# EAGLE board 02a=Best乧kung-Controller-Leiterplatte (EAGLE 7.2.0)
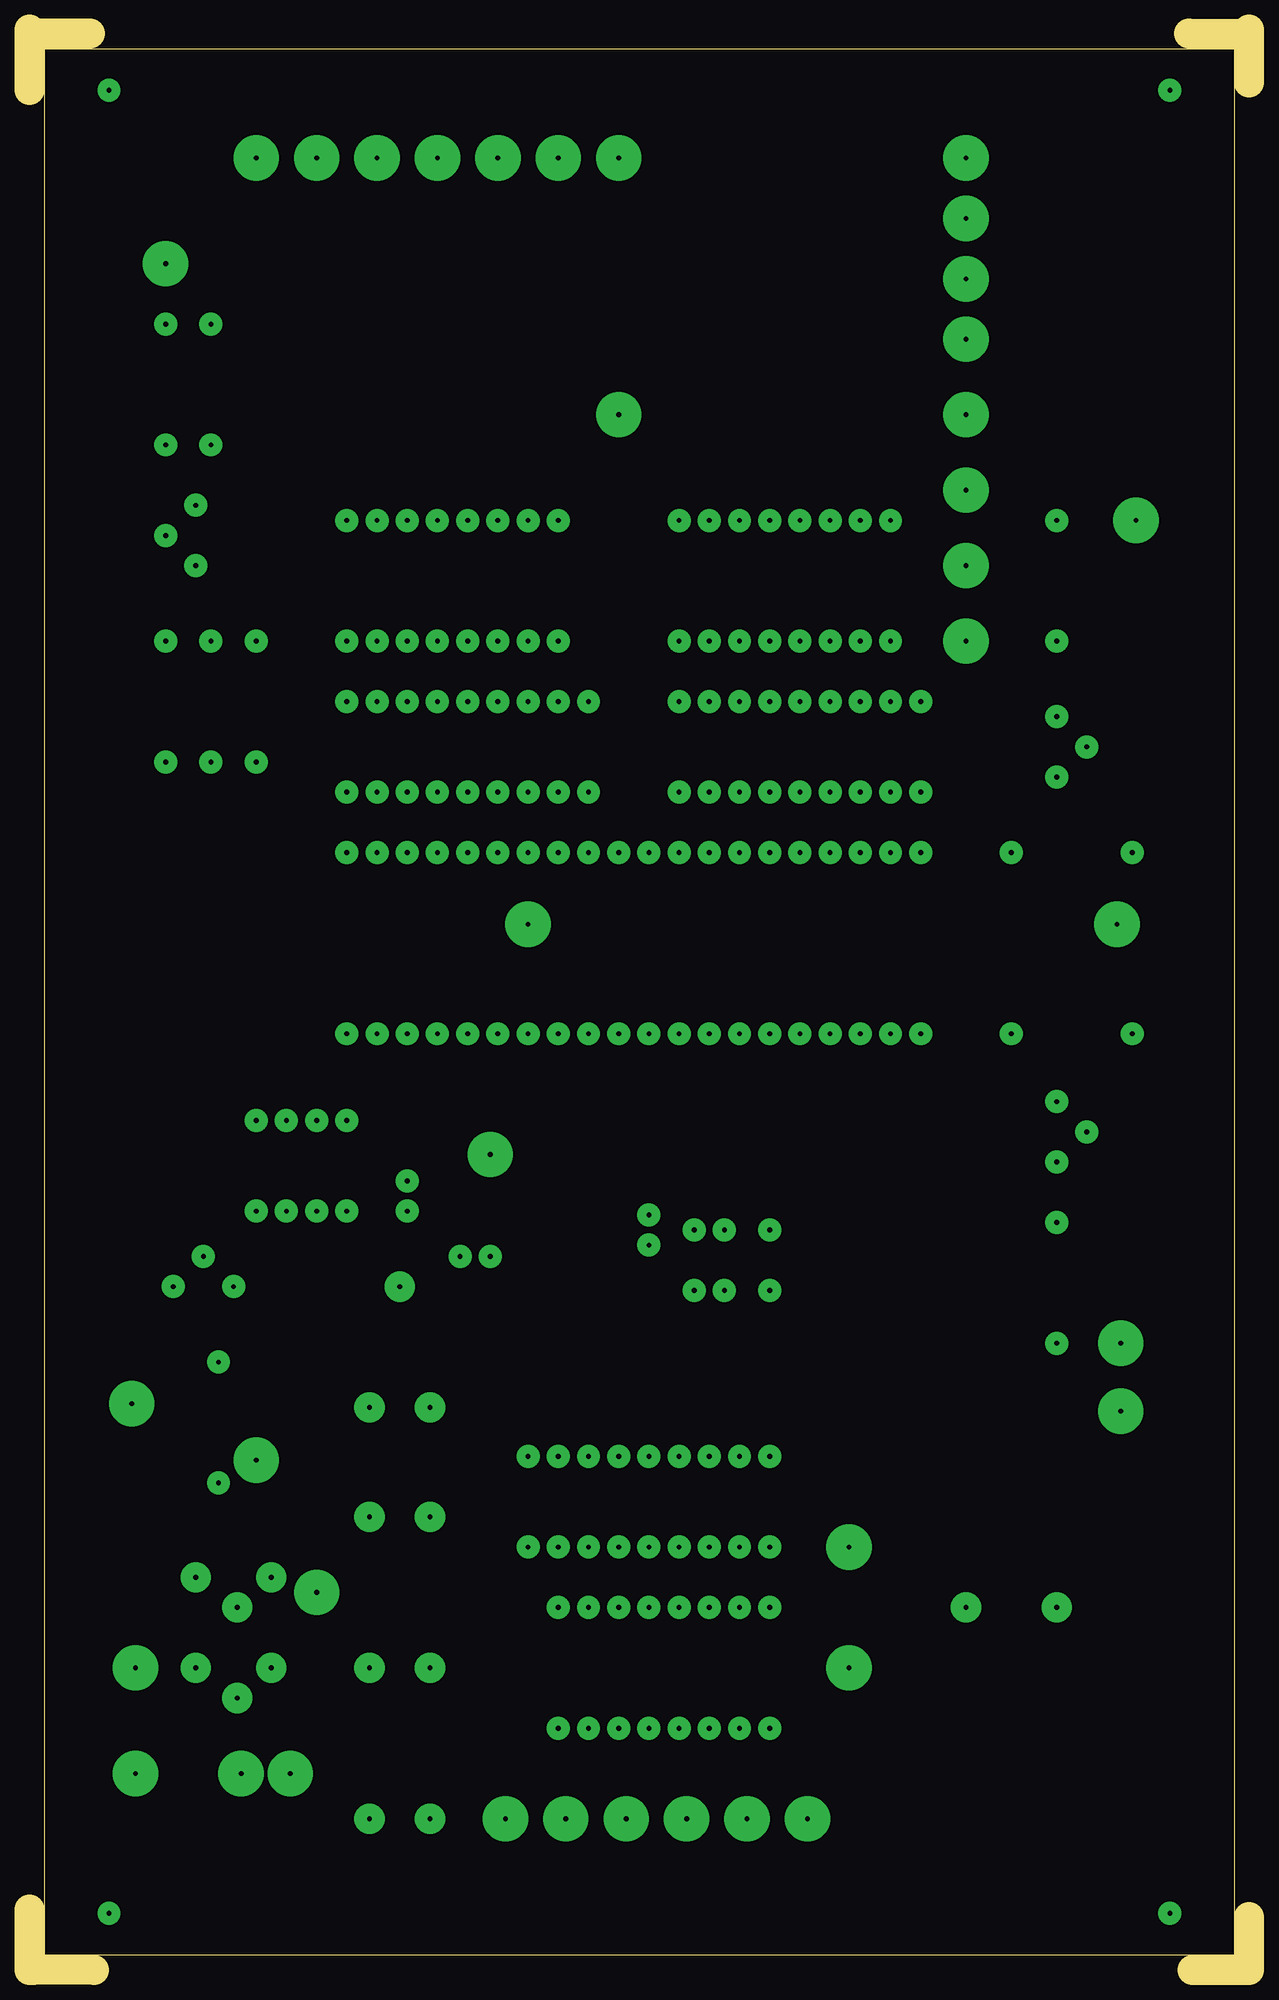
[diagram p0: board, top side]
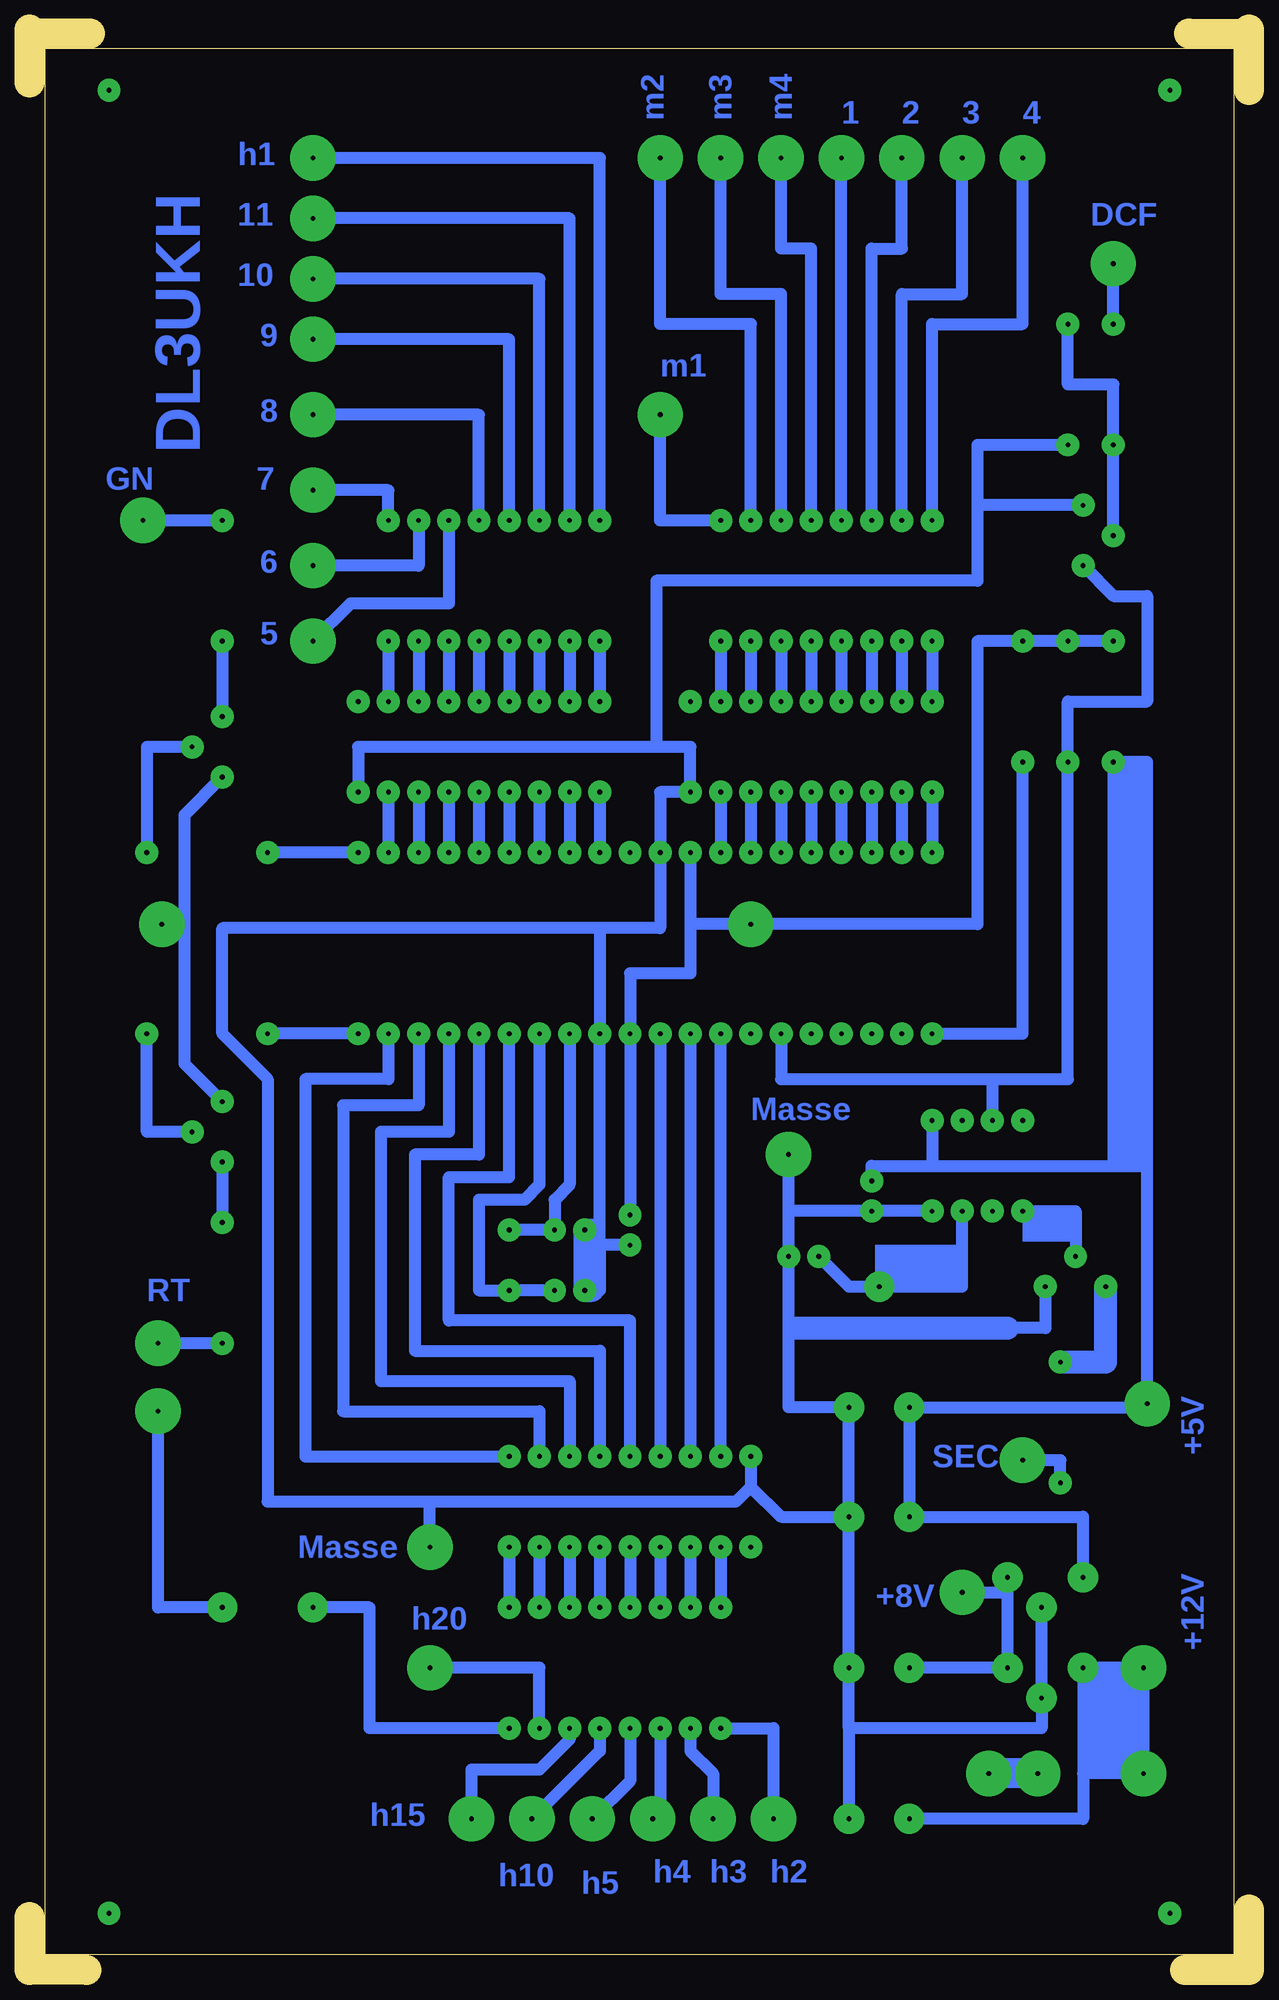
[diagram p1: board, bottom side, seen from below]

Size 102.55 x 163.2 mm. Coordinates in mm from the lower left corner, seen from the top.
Outline: 5.4,0 0.32,0
Outline: 0,0 0,5.08
Outline: 97.79,0 102.55,0 102.55,4.45
Outline: 5.08,162.88 0,162.88
Outline: 0,158.12 0,162.88
Outline: 0,162.88 0,163.2
Outline: 102.55,158.75 102.55,163.2
Outline: 97.47,162.88 102.23,162.88
Outline: 1.27,1.27 101.28,1.27 101.28,161.61 1.27,161.61 1.27,1.27
Copper layers (1*16): Top 0.035mm / dielectric 1.5mm / Bottom 0.035mm
Design rules "default": minimum track width 10mil, minimum drill 24mil, track to track 8mil, track to pad 8mil, pad to pad 8mil, via to via 8mil, smd to smd 8mil, copper to edge 40mil, drill to drill 8mil, minimum pad ring 10mil, minimum via ring 8mil, stop-mask expansion 4mil, vias tented up to drill 0mil, thermal gap 10mil

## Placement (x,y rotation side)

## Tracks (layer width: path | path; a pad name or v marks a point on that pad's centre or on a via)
S$1  (via drill 0.4 pad 1.93, 0.4 pad 3.81)
  Bottom 1.016: v26.67,121.92 26.67,138.43 19.05,138.43 v19.05,152.4 19.05,152.72
S$2  (via drill 0.4 pad 1.93)
  Bottom 1.016: v54.61,99.06 v54.61,93.98
S$3  (via drill 0.4 pad 1.93)
  Bottom 1.016: v57.15,99.06 v57.15,93.98
S$4  (via drill 0.4 pad 1.93)
  Bottom 1.016: v59.69,99.06 v59.69,93.98
S$5  (via drill 0.4 pad 1.93)
  Bottom 1.016: v62.23,99.06 v62.23,93.98
S$6  (via drill 0.4 pad 1.93)
  Bottom 1.016: v64.77,99.06 v64.77,93.98
S$7  (via drill 0.4 pad 1.93)
  Bottom 1.016: v67.31,99.06 v67.31,93.98
S$8  (via drill 0.4 pad 1.93)
  Bottom 1.016: v69.85,99.06 v69.85,93.98
S$9  (via drill 0.4 pad 1.93)
  Bottom 1.016: v72.39,99.06 v72.39,93.98
S$10  (via drill 0.4 pad 2.54, 0.4 pad 3.81)
  Bottom 1.016: v28.57,25.4 v20.32,25.4 20.32,31.75 | 20.32,31.75 v20.32,33.02 | v24.13,31.75 20.32,31.75
S$11  (via drill 0.4 pad 1.93, 0.4 pad 3.81)
  Bottom 1.016: v69.85,121.92 69.85,118.11 v78.74,118.11
S$12  (via drill 0.4 pad 1.93)
  other vias: 95.88,4.76
S$13  (via drill 0.4 pad 3.81)
  Bottom 2.54: v17.78,16.51 v21.91,16.51
S$14  (via drill 0.4 pad 1.93)
  other vias: 31.75,78.74
S$15  (via drill 0.4 pad 2.54)
  Bottom 1.016: 28.57,47.31 v28.57,38.1 13.97,38.1 v13.97,33.02
S$16  (via drill 0.4 pad 1.93)
  other vias: 36.83,78.74
S$17  (via drill 0.4 pad 1.93, 0.4 pad 2.54, 0.4 pad 3.81)
  Bottom 1.016: v59.69,20.32 59.69,25.4 v68.9,25.4 | v13.97,123.19 22.86,123.19 | 22.86,123.19 22.86,116.84 49.85,116.84 49.85,102.87 | v41.91,43.18 41.91,40.64 | 41.91,40.64 39.37,38.1 v33.66,38.1 | 33.66,20.32 17.46,20.32 v17.46,22.86 17.46,30.48 | v33.66,38.1 v33.66,25.4 33.66,20.32 | 33.66,20.32 v33.66,12.7 | 41.91,40.64 43.18,39.37 68.9,39.37 | 68.9,39.37 82.55,39.37 82.55,74.93 86.36,78.74 86.36,87.63 54.61,87.63 | 38.74,53.98 38.74,47.31 v33.66,47.31 v33.66,38.1 | 38.74,53.98 v38.74,60.01 38.74,68.58 | v17.14,57.47 17.14,53.98 20.32,53.98 | 38.1,53.98 38.74,53.98 | v74.93,99.06 74.93,102.87 49.85,102.87 | 49.85,102.87 46.99,102.87 v46.99,99.06 49.53,99.06 v49.53,93.98 49.53,87.63 54.61,87.63 | 54.61,87.63 v54.61,78.74 54.61,60.96 | v52.07,60.96 54.61,60.96 | 54.61,60.96 54.61,57.15 55.25,57.15 | v15.24,128.27 22.86,128.27 22.86,123.19 | v68.9,35.56 68.9,39.37
  Bottom 1.93: 38.1,53.98 20.32,53.98 | 55.25,62.23 v55.88,62.23 v55.88,57.15 55.25,57.15
S$18  (via drill 0.4 pad 1.93)
  other vias: 41.91,78.74
S$19  (via drill 0.4 pad 1.93)
  other vias: 29.21,78.74
S$20  (via drill 0.4 pad 1.93)
  Bottom 1.016: v46.99,78.74 v46.99,43.18
S$21  (via drill 0.4 pad 1.93)
  Bottom 1.016: v49.53,78.74 v49.53,43.18
S$22  (via drill 0.4 pad 1.93)
  other vias: 52.07,93.98
S$23  (via drill 0.4 pad 1.93)
  other vias: 74.93,106.68
S$24  (via drill 0.4 pad 1.93)
  other vias: 82.55,93.98
S$25  (via drill 0.4 pad 1.93, 0.4 pad 3.81)
  Bottom 1.016: v86.36,100.33 89.53,97.16 89.53,87.95 | 89.53,87.95 89.53,76.2 v86.36,73.02 | v91.44,87.95 89.53,87.95
  other vias: 38.74,68.58 41.91,87.95
S$26  (via drill 0.4 pad 1.93)
  other vias: 34.29,78.74
S$27  (via drill 0.4 pad 1.93)
  Bottom 1.016: v26.67,78.74 19.05,78.74 v19.05,101.6
S$28  (via drill 0.4 pad 2.54, 0.4 pad 3.81)
  Bottom 1.016: v28.57,12.7 13.97,12.7 13.97,16.51 | 13.97,16.51 v13.97,25.4 v8.89,25.4 v8.89,16.51 13.97,16.51
S$29  (via drill 0.4 pad 1.93)
  Bottom 1.016: v86.36,67.94 v86.36,62.87
S$30  (via drill 0.4 pad 1.93)
  Bottom 1.016: v88.9,70.48 92.71,70.48 v92.71,78.74
S$31  (via drill 0.4 pad 1.93)
  Bottom 1.016: v74.93,93.98 82.87,93.98
S$33  (via drill 0.4 pad 1.93, 0.4 pad 3.81)
  Bottom 1.016: v86.36,52.71 v91.76,52.71
S$34  (via drill 0.4 pad 1.93)
  Bottom 1.016: v57.15,78.74 57.15,66.04 58.42,64.77 v58.42,62.23 v62.23,62.23
S$35  (via drill 0.4 pad 1.93)
  Bottom 1.016: v59.69,78.74 59.69,66.04 60.96,64.77 64.77,64.77 64.77,57.15 v62.23,57.15 v58.42,57.15
S$36  (via drill 0.4 pad 1.93, 0.4 pad 3.81)
  Bottom 1.016: v15.88,40.96 15.88,42.86 v19.05,42.86
S$37  (via drill 0.4 pad 1.93)
  Bottom 1.016: v64.77,78.74 64.77,68.58 70.17,68.58 70.17,52.07 54.61,52.07 v54.61,43.18
S$38  (via drill 0.4 pad 1.93)
  Bottom 1.016: v67.31,78.74 67.31,70.48 73.02,70.48 73.02,49.53 57.15,49.53 v57.15,43.18
S$39  (via drill 0.4 pad 1.93)
  Bottom 1.016: v69.85,78.74 69.85,72.71 76.2,72.71 76.2,46.99 59.69,46.99 v59.69,43.18
S$40  (via drill 0.4 pad 1.93)
  Bottom 1.016: v72.39,78.74 72.39,74.93 79.38,74.93 79.38,43.18 v62.23,43.18
S$41  (via drill 0.4 pad 1.93)
  Bottom 1.016: v74.93,78.74 v82.55,78.74
S$42  (via drill 0.4 pad 1.93)
  Bottom 1.016: v26.67,99.06 v26.67,93.98
S$43  (via drill 0.4 pad 1.93)
  Bottom 1.016: v29.21,99.06 v29.21,93.98
S$44  (via drill 0.4 pad 1.93)
  Bottom 1.016: v31.75,99.06 v31.75,93.98
S$45  (via drill 0.4 pad 1.93)
  Bottom 1.016: v34.29,99.06 v34.29,93.98
S$46  (via drill 0.4 pad 1.93)
  Bottom 1.016: v36.83,99.06 v36.83,93.98
S$47  (via drill 0.4 pad 1.93)
  Bottom 1.016: v39.37,99.06 v39.37,93.98
S$48  (via drill 0.4 pad 1.93)
  Bottom 1.016: v41.91,99.06 v41.91,93.98
S$49  (via drill 0.4 pad 1.93)
  Bottom 1.016: v44.45,99.06 v44.45,93.98
S$50  (via drill 0.4 pad 2.54)
  other vias: 17.46,30.48
S$51  (via drill 0.4 pad 1.93, 0.4 pad 3.81)
  Bottom 1.016: v52.07,20.32 52.07,15.88 v55.25,12.7
S$52  (via drill 0.4 pad 1.93, 0.4 pad 3.81)
  Bottom 1.016: v29.21,121.92 29.21,140.97 24.13,140.97 v24.13,152.4
S$53  (via drill 0.4 pad 1.93)
  other vias: 31.75,106.68
S$54  (via drill 0.4 pad 1.93)
  other vias: 34.29,106.68
S$55  (via drill 0.4 pad 1.93)
  Bottom 1.016: v52.07,63.5 v52.07,78.74 52.07,83.82 46.99,83.82 46.99,87.95 | v46.99,93.98 46.99,87.95 | 46.99,87.95 22.86,87.95 22.86,111.76 v19.05,111.76 v15.24,111.76 v11.43,111.76
S$56  (via drill 0.4 pad 1.93, 0.4 pad 3.81)
  Bottom 1.016: v45.09,12.7 45.09,16.51 46.99,18.41 v46.99,20.32
S$57  (via drill 0.4 pad 1.93, 0.4 pad 3.81)
  Bottom 1.016: v57.15,20.32 57.15,19.37 59.69,16.83 65.41,16.83 65.41,15.88 65.41,15.56 v65.41,12.7
S$58  (via drill 0.4 pad 1.93, 0.4 pad 3.81)
  Bottom 1.016: v49.53,20.32 49.53,13.33 v50.17,12.7
S$59  (via drill 0.4 pad 1.93)
  Bottom 1.016: v88.9,102.87 92.71,102.87 v92.71,93.98
S$60  (via drill 0.4 pad 1.93, 0.4 pad 3.81)
  Bottom 1.016: v54.61,20.32 54.61,18.41 v60.33,12.7
S$61  (via drill 0.4 pad 1.93)
  other vias: 41.91,35.56
S$62  (via drill 0.4 pad 1.93)
  Bottom 1.016: v44.45,35.56 v44.45,30.48
S$63  (via drill 0.4 pad 1.93)
  Bottom 1.016: v46.99,35.56 v46.99,30.48
S$64  (via drill 0.4 pad 1.93)
  Bottom 1.016: v49.53,35.56 v49.53,30.48
S$65  (via drill 0.4 pad 1.93)
  Bottom 1.016: v52.07,35.56 v52.07,30.48
S$66  (via drill 0.4 pad 1.93)
  Bottom 1.016: v54.61,35.56 v54.61,30.48
S$67  (via drill 0.4 pad 1.93)
  Bottom 1.016: v57.15,35.56 v57.15,30.48
S$68  (via drill 0.4 pad 1.93)
  Bottom 1.016: v59.69,35.56 v59.69,30.48
S$69  (via drill 0.4 pad 1.93)
  Bottom 1.016: v62.23,35.56 v62.23,30.48
S$71  (via drill 0.4 pad 1.93)
  Bottom 1.016: v44.45,43.18 v44.45,78.74
S$72  (via drill 0.4 pad 1.93)
  Bottom 1.016: v86.36,111.76 v86.36,105.41
S$73  (via drill 0.4 pad 1.93, 0.4 pad 3.81)
  Bottom 1.016: v86.36,121.92 v93.03,121.92
S$74  (via drill 0.4 pad 1.93)
  Bottom 1.016: v52.07,43.18 52.07,54.61 67.31,54.61 67.31,66.67 62.23,66.67 v62.23,78.74
S$75  (via drill 0.4 pad 1.93)
  Bottom 1.016: v26.67,111.76 v26.67,106.68
S$76  (via drill 0.4 pad 1.93)
  Bottom 1.016: v29.21,111.76 v29.21,106.68
S$77  (via drill 0.4 pad 1.93)
  Bottom 1.016: v31.75,111.76 31.75,106.36
S$78  (via drill 0.4 pad 1.93)
  Bottom 1.016: v34.29,111.76 34.29,106.36
S$80  (via drill 0.4 pad 2.54, 0.4 pad 3.81)
  Bottom 1.016: v86.36,30.48 91.76,30.48 v91.76,46.99
S$81  (via drill 0.4 pad 1.93, 0.4 pad 3.81)
  Bottom 1.016: v11.43,138.43 v11.43,143.51
S$82  (via drill 0.4 pad 1.93)
  other vias: 6.67,4.76
S$83  (via drill 0.4 pad 1.93)
  other vias: 6.67,158.12
S$86  (via drill 0.4 pad 1.93)
  Bottom 1.016: v36.83,111.76 v36.83,106.68
S$87  (via drill 0.4 pad 1.93)
  other vias: 46.99,106.68
S$88  (via drill 0.4 pad 1.93)
  Bottom 1.016: v39.37,111.76 v39.37,106.68
S$89  (via drill 0.4 pad 1.93)
  Bottom 1.016: v41.91,111.76 v41.91,106.68
S$90  (via drill 0.4 pad 1.93)
  Bottom 1.016: v44.45,111.76 v44.45,106.68
S$91  (via drill 0.4 pad 1.93)
  Bottom 1.016: v54.61,111.76 v54.61,106.68
S$92  (via drill 0.4 pad 1.93)
  Bottom 1.016: v57.15,111.76 v57.15,106.68
S$93  (via drill 0.4 pad 1.93)
  Bottom 1.016: v59.69,111.76 v59.69,106.68
S$94  (via drill 0.4 pad 1.93)
  Bottom 1.016: v62.23,111.76 v62.23,106.68
S$95  (via drill 0.4 pad 1.93)
  Bottom 1.016: v64.77,111.76 v64.77,106.68
S$96  (via drill 0.4 pad 1.93)
  Bottom 1.016: v67.31,111.76 v67.31,106.68
S$97  (via drill 0.4 pad 1.93)
  Bottom 1.016: v69.85,111.76 v69.85,106.68
S$98  (via drill 0.4 pad 1.93)
  Bottom 1.016: v72.39,111.76 v72.39,106.68
S$101  (via drill 0.4 pad 1.93, 0.4 pad 3.81)
  Bottom 1.016: v31.75,121.92 31.75,144.78 29.21,144.78 v29.21,152.4
S$102  (via drill 0.4 pad 1.93, 0.4 pad 3.81)
  Bottom 1.016: v34.29,121.92 v34.29,152.4
S$103  (via drill 0.4 pad 1.93, 0.4 pad 3.81)
  Bottom 1.016: v36.83,121.92 36.83,144.78 39.37,144.78 v39.37,152.4
S$104  (via drill 0.4 pad 1.93, 0.4 pad 3.81)
  Bottom 1.016: v39.37,121.92 39.37,140.97 44.45,140.97 v44.45,152.4
S$105  (via drill 0.4 pad 1.93, 0.4 pad 3.81)
  Bottom 1.016: v41.91,121.92 41.91,138.43 49.53,138.43 49.53,152.08 v49.53,152.4
S$106  (via drill 0.4 pad 1.93, 0.4 pad 3.81)
  Bottom 1.016: v44.45,121.92 49.53,121.92 v49.53,130.81
S$107  (via drill 0.4 pad 1.93, 0.4 pad 3.81)
  Bottom 1.016: v54.61,121.92 54.61,152.4 v78.74,152.4
S$108  (via drill 0.4 pad 1.93, 0.4 pad 3.81)
  Bottom 1.016: v57.15,121.92 57.15,147.32 v78.74,147.32
S$109  (via drill 0.4 pad 1.93, 0.4 pad 3.81)
  Bottom 1.016: v59.69,121.92 59.69,142.24 v78.74,142.24
S$110  (via drill 0.4 pad 1.93, 0.4 pad 3.81)
  Bottom 1.016: v62.23,121.92 62.23,137.16 v78.74,137.16
S$111  (via drill 0.4 pad 1.93, 0.4 pad 3.81)
  Bottom 1.016: v64.77,121.92 64.77,130.81 v78.74,130.81
S$112  (via drill 0.4 pad 1.93, 0.4 pad 3.81)
  Bottom 1.016: v67.31,121.92 67.31,114.94 75.56,114.94 v78.74,111.76
S$113  (via drill 0.4 pad 1.93)
  other vias: 95.88,158.12
S$114  (via drill 0.4 pad 1.93, 0.4 pad 3.81)
  Bottom 1.016: v72.39,121.92 72.39,124.46 v78.74,124.46
S$117  (via drill 0.4 pad 1.93)
  Bottom 1.016: v13.97,118.11 11.43,115.57 8.57,115.57 8.57,106.68 15.24,106.68 v15.24,101.6 15.24,74.93 21.59,74.93 | v39.37,78.74 39.37,74.93 21.59,74.93 | 21.59,74.93 v21.59,71.44
S$119  (via drill 0.4 pad 1.93)
  Bottom 1.016: v11.43,120.65 v11.43,128.27 11.43,133.35 15.24,133.35 v15.24,138.43
S$123  (via drill 0.4 pad 1.93, 0.4 pad 3.81)
  Bottom 1.016: v44.45,20.32 40.01,20.32 v40.01,12.7
S$128  (via drill 0.4 pad 1.93)
  other vias: 24.13,71.44
S$129  (via drill 0.4 pad 1.93)
  other vias: 19.05,71.44
S$130  (via drill 0.4 pad 1.93, 0.4 pad 2.54)
  Bottom 1.016: v62.23,20.32 73.98,20.32 73.98,30.48 v78.74,30.48
S$131  (via drill 0.4 pad 1.93)
  Bottom 1.016: v19.05,63.82 14.61,63.82 v14.61,60.01
S$132  (via drill 0.4 pad 1.93)
  other vias: 21.59,63.82
S$133  (via drill 0.4 pad 1.93)
  Bottom 1.016: v26.67,63.82 v31.75,63.82 38.74,63.82
S$134  (via drill 0.4 pad 1.93, 0.4 pad 2.54)
  Bottom 1.016: v24.13,63.82 24.13,57.47 v31.11,57.47 33.66,57.47 v36.2,60.01
S$135  (via drill 0.4 pad 1.93)
  Bottom 1.93: v15.88,51.12 12.06,51.12 v12.06,57.47
S$138  (via drill 0.4 pad 1.93, 0.4 pad 2.54, 0.4 pad 3.81)
  Bottom 1.016: v28.57,47.31 8.57,47.31 v8.57,47.62 8.57,67.63 | v26.67,71.44 26.67,67.63 | 26.67,67.63 8.57,67.63 | v31.75,66.36 31.75,67.63 26.67,67.63 | 8.57,67.63 8.57,101.6 v11.43,101.6 11.43,67.94
(copper drawn outside any net)
  shapes: Bottom area x5

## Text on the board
Bottom: 4 | 3 | 2 | 1 | m4 | m3 | m2 | h1 | DL3UKH | DCF | 11 | 10 | 9 | m1 | 8 | 7 | GN | 6 | 5 | Masse | RT | +5V | SEC | Masse | +12V | +8V | h20 | h15 | h2 | h3 | h4 | h10 | h5
Vias: Auf Bestückungsseite gesehen !
Dimension: K
tOrigins: µA78L05 und µA78L05 | BC547c und BC557c | 2N7000 | Ausg. | Eing. | C | E | S | D | G | B | Masse | IC's | 750K | 220K | 1 | 1N4002 | Die Aussparung | BC547c | Links oben ist | muß mit dem | E | immer PIN 1 | Bauelement | und dem Bestück- | Widerstände | ungsplan | K | siehe Stromlaufplan | überein stimmen. | 180 | Katode | Anode | BC557c | K | Br. | 10K | 10K | ULN2803A | ULN2803A | 1 | 1 | E | Leiterplatte: | 1,5mm dick | Br. | 12K | Cevausit | Alles mit 0,8mm vorbohren ! | PIC16F877A | Aufbohren: | 1 | 12K | Diode 1N4002 1,0mm | BC557c | E | Einstellregler 1,2mm | 1 | vielleicht 4Stck. Befestigungsbohr... 3,2mm | PIC12F675 | K | 2N7000 | 15p | 47n | G | 47n | 47n | D | 16Mhz | S | nicht vergessen ! | 180 | Die zwei Brücken (Br.) | 15p | Eine Brücke ist unter der großen IC-Fassung ! | 5K | +5V | 180 | Steht für den | + | 1 | Pluspol eines | ULN2803A | Ausg. | Elkos | 470µ/35V | + | - | + ist immer | µA78L05 | Widerstände | langer Draht | + | Ausg. | siehe Stromlaufplan | Summer | µA78L08 | 470µ/35V | hier an LED-Leiterpl. | also die +12V | +12vEing. | Schalter / danach an +5Volt | + | K | 1N4002 | 470µ/35V | hier +12V vom Steckernetzteil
